[IBIS Ver]   5.1
[File name]   imx8mm_14x14_v1.ibs
[File Rev]   1.0
[Date]   Jan 06,2021
[Notes]   One-Section RLC
[Disclaimer] IMPORTANT NOTICE
  This information is provided on an AS IS basis and without warranty.
  IN NO EVENT SHALL NXP BE LIABLE FOR INCIDENTAL OR CONSEQUENTIAL
  DAMAGES ARISING FROM USE OF THIS INFORMATION. THIS DISCLAIMER OF
  WARRANTY EXTENDS TO THE USER OF THE INFORMATION, AND TO THEIR CUSTOMERS
  OR USERS OF PRODUCTS  AND IS IN LIEU OF ALL WARRANTIES WHETHER EXPRESS,
  IMPLIED, OR STATUTORY, INCLUDING IMPLIED WARRANTIES OF MERCHANTABILITY
  OR FITNESS FOR PARTICULAR PURPOSE.
  NXP does not represent or warrant that the information furnished
  hereunder is free of infringement of any third party patents,
  copyrights, trade secrets, or other intellectual property rights.
  NXP does not represent or warrant that the information is free of
  defect, or that it meets any particular standard, requirements or need
  of the user of the infomation or their customers.
  NXP reserves the right to change the information in this file
  without notice.
   http://www.nxp.com
[Copyright]   (C) Copyright NXP 2007 - 2018, All Rights Reserved.
[Component] imx8mm_14x14_v1.ibs
[Manufacturer] NXP
[Package]
|   typ   min   max
R_pkg   0.37144   0.16325   0.62648
L_pkg   2.82e-9   1.063e-9   4.842e-9
C_pkg   7.818e-13   4.515e-13   1.089e-12
[Pin]   Signal_name   model_name   R_pin   L_pin   C_pin
M19 NVCC_CLK POWER
K8 NVCC_DRAM POWER
K9 NVCC_DRAM POWER
L9 NVCC_DRAM POWER
M9 NVCC_DRAM POWER
N8 NVCC_DRAM POWER
N9 NVCC_DRAM POWER
P7 NVCC_DRAM POWER
R8 NVCC_DRAM POWER
R9 NVCC_DRAM POWER
T9 NVCC_DRAM POWER
U9 NVCC_DRAM POWER
V8 NVCC_DRAM POWER
V9 NVCC_DRAM POWER
H10 NVCC_ECSPI POWER
W22 NVCC_ENET POWER
W12 NVCC_GPIO1 POWER
J11 NVCC_I2C POWER
L19 NVCC_JTAG POWER
U19 NVCC_NAND POWER
W18 NVCC_SAI1 POWER
V19 NVCC_SAI2 POWER
Y10 NVCC_SAI3 POWER
W17 NVCC_SAI5 POWER
V20 NVCC_SD1 POWER
V22 NVCC_SD2 POWER
J22 NVCC_SNVS_1P8 POWER
J12 NVCC_UART POWER
AB13 PVCC0_1P8 POWER
T19 PVCC1_1P8 POWER
J13 PVCC2_1P8 POWER
N19 VDD_24M_XTAL_1P8 POWER
AA14 VDD_ANA0_1P8 POWER
Y15 VDD_ANA0_1P8 POWER
N20 VDD_ANA1_1P8 POWER
P19 VDD_ANA1_1P8 POWER
L17 VDD_ANA_0P8 POWER
N17 VDD_ANA_0P8 POWER
R13 VDD_ARM POWER
R15 VDD_ARM POWER
T13 VDD_ARM POWER
T14 VDD_ARM POWER
T15 VDD_ARM POWER
U13 VDD_ARM POWER
U15 VDD_ARM POWER
V13 VDD_ARM POWER
V15 VDD_ARM POWER
V16 VDD_ARM POWER
W13 VDD_ARM POWER
W14 VDD_ARM POWER
W15 VDD_ARM POWER
W16 VDD_ARM POWER
P16 VDD_ARM_PLL_0P8 POWER
R19 VDD_ARM_PLL_1P8 POWER
J10 VDD_DRAM POWER
L10 VDD_DRAM POWER
N10 VDD_DRAM POWER
R10 VDD_DRAM POWER
U10 VDD_DRAM POWER
W10 VDD_DRAM POWER
P9 VDD_DRAM_PLL_0P8 POWER
P5 VDD_DRAM_PLL_1P8 POWER
P12 VDD_GPU POWER
R11 VDD_GPU POWER
U11 VDD_GPU POWER
V12 VDD_GPU POWER
W11 VDD_GPU POWER
J14 VDD_MIPI_0P9 POWER
J15 VDD_MIPI_1P2 POWER
H13 VDD_MIPI_1P8 POWER
J16 VDD_PCI_0P8 POWER
G14 VDD_PCI_1P8 POWER
K22 VDD_SNVS_0P8 POWER
K15 VDD_SOC POWER
K16 VDD_SOC POWER
L15 VDD_SOC POWER
L18 VDD_SOC POWER
M15 VDD_SOC POWER
N13 VDD_SOC POWER
N15 VDD_SOC POWER
N18 VDD_SOC POWER
R17 VDD_SOC POWER
R18 VDD_SOC POWER
U17 VDD_SOC POWER
U18 VDD_SOC POWER
J17 VDD_USB_0P8 POWER
H15 VDD_USB_1P8 POWER
K19 VDD_USB_3P3 POWER
K12 VDD_VPU POWER
K13 VDD_VPU POWER
L11 VDD_VPU POWER
L13 VDD_VPU POWER
M13 VDD_VPU POWER
M14 VDD_VPU POWER
N11 VDD_VPU POWER
P1 DRAM_VREF POWER
B27 24M_XTALI NC 0.4921 3.82E-09 9.28E-13
C26 24M_XTALO NC 0.45748 3.59E-09 8.46E-13
G26 BOOT_MODE0 PBIDIRHS_E33_33_NT_DR_H 0.38307 3.00E-09 8.24E-13
G27 BOOT_MODE1 PBIDIRHS_E33_33_NT_DR_H 0.40036 3.16E-09 8.38E-13
H27 CLKIN1 PBIDIRHS_E33_33_NT_DR_H 0.36937 3.01E-09 8.01E-13
J27 CLKIN2 PBIDIRHS_E33_33_NT_DR_H 0.4193 3.52E-09 8.49E-13
H26 CLKOUT1 PBIDIRHS_E33_33_NT_DR_H 0.35917 2.90E-09 8.78E-13
J26 CLKOUT2 PBIDIRHS_E33_33_NT_DR_H 0.42161 3.44E-09 8.89E-13
F4 DRAM_AC00 CA_CK 0.42341 3.09E-09 8.52E-13
F5 DRAM_AC01 CA_CK 0.29473 2.13E-09 7.50E-13
K4 DRAM_AC02 CA_CK 0.3399 2.45E-09 5.61E-13
J4 DRAM_AC03 CA_CK 0.36868 2.58E-09 7.56E-13
L2 DRAM_AC04 CA_CK 0.33939 2.34E-09 7.22E-13
L1 DRAM_AC05 CA_CK 0.34212 2.36E-09 7.20E-13
F6 DRAM_AC06 CA_CK 0.34818 2.62E-09 8.00E-13
J5 DRAM_AC07 CA_CK 0.26386 1.87E-09 6.85E-13
J6 DRAM_AC08 CA_CK 0.31308 2.36E-09 6.60E-13
K6 DRAM_AC09 CA_CK 0.20679 1.49E-09 5.66E-13
E4 DRAM_AC10 CA_CK 0.41222 3.00E-09 9.97E-13
D5 DRAM_AC11 CA_CK 0.47769 3.53E-09 1.01E-12
N4 DRAM_AC12 CA_CK 0.24984 1.70E-09 6.69E-13
N5 DRAM_AC13 CA_CK 0.284 1.98E-09 5.24E-13
K5 DRAM_AC14 CA_CK 0.34768 2.50E-09 7.57E-13
N6 DRAM_AC15 CA_CK 0.16325 1.06E-09 4.70E-13
M1 DRAM_AC16 CA_CK 0.31836 2.25E-09 6.88E-13
M2 DRAM_AC17 CA_CK 0.32445 2.22E-09 6.95E-13
N2 DRAM_AC19 CA_CK 0.34499 2.50E-09 7.43E-13
AB4 DRAM_AC20 CA_CK 0.37465 2.80E-09 9.48E-13
AB5 DRAM_AC21 CA_CK 0.38319 2.90E-09 9.15E-13
W4 DRAM_AC22 CA_CK 0.38211 2.84E-09 8.08E-13
V4 DRAM_AC23 CA_CK 0.29471 2.10E-09 7.54E-13
U2 DRAM_AC24 CA_CK 0.34737 2.38E-09 7.32E-13
U1 DRAM_AC25 CA_CK 0.34266 2.43E-09 7.32E-13
N1 DRAM_AC26 CA_CK 0.42632 3.11E-09 9.15E-13
R6 DRAM_AC27 CA_CK 0.22559 1.66E-09 5.07E-13
W6 DRAM_AC28 CA_CK 0.22056 1.60E-09 6.33E-13
V6 DRAM_AC29 CA_CK 0.27799 1.96E-09 6.03E-13
AC4 DRAM_AC30 CA_CK 0.48641 3.58E-09 9.77E-13
AD5 DRAM_AC31 CA_CK 0.41562 3.11E-09 1.02E-12
R4 DRAM_AC32 CA_CK 0.2504 1.78E-09 6.58E-13
R5 DRAM_AC33 CA_CK 0.33425 2.46E-09 6.16E-13
T1 DRAM_AC34 CA_CK 0.321 2.31E-09 7.99E-13
T2 DRAM_AC35 CA_CK 0.42263 2.99E-09 8.89E-13
V5 DRAM_AC36 CA_CK 0.2084 1.47E-09 4.76E-13
W5 DRAM_AC37 CA_CK 0.2624 1.85E-09 6.65E-13
AB6 DRAM_AC38 CA_CK 0.34026 2.47E-09 7.31E-13
R2 DRAM_ALERT_N CA_CK 0.27399 1.90E-09 6.80E-13
A4 DRAM_DM0 DQ_DQS 0.47819 3.40E-09 9.75E-13
F1 DRAM_DM1 DQ_DQS 0.49651 3.45E-09 9.97E-13
AB1 DRAM_DM2 DQ_DQS 0.48699 3.28E-09 8.55E-13
AG4 DRAM_DM3 DQ_DQS 0.43626 2.94E-09 9.57E-13
A5 DRAM_DQ00 DQ_DQS 0.38783 2.72E-09 8.18E-13
B5 DRAM_DQ01 DQ_DQS 0.36282 2.46E-09 7.49E-13
D2 DRAM_DQ02 DQ_DQS 0.4521 3.16E-09 9.42E-13
D1 DRAM_DQ03 DQ_DQS 0.41453 2.88E-09 9.24E-13
C1 DRAM_DQ04 DQ_DQS 0.5585 3.72E-09 9.55E-13
B1 DRAM_DQ05 DQ_DQS 0.50545 3.31E-09 1.01E-12
A3 DRAM_DQ06 DQ_DQS 0.5562 3.84E-09 1.09E-12
B4 DRAM_DQ07 DQ_DQS 0.38982 2.83E-09 9.33E-13
F2 DRAM_DQ08 DQ_DQS 0.38671 2.53E-09 7.96E-13
G2 DRAM_DQ09 DQ_DQS 0.43825 3.05E-09 7.98E-13
J1 DRAM_DQ10 DQ_DQS 0.34914 2.55E-09 8.27E-13
J2 DRAM_DQ11 DQ_DQS 0.40764 2.85E-09 7.90E-13
K2 DRAM_DQ12 DQ_DQS 0.32705 2.20E-09 7.37E-13
K1 DRAM_DQ13 DQ_DQS 0.4328 2.98E-09 8.00E-13
E1 DRAM_DQ14 DQ_DQS 0.43043 3.20E-09 1.07E-12
E2 DRAM_DQ15 DQ_DQS 0.39934 2.85E-09 9.64E-13
AB2 DRAM_DQ16 DQ_DQS 0.39751 2.80E-09 9.41E-13
AA2 DRAM_DQ17 DQ_DQS 0.42671 3.06E-09 8.23E-13
W1 DRAM_DQ18 DQ_DQS 0.45851 3.22E-09 9.25E-13
W2 DRAM_DQ19 DQ_DQS 0.35718 2.37E-09 7.42E-13
V2 DRAM_DQ20 DQ_DQS 0.42378 2.95E-09 9.70E-13
V1 DRAM_DQ21 DQ_DQS 0.40154 2.74E-09 9.04E-13
AC1 DRAM_DQ22 DQ_DQS 0.50433 3.37E-09 8.78E-13
AC2 DRAM_DQ23 DQ_DQS 0.39804 2.61E-09 8.82E-13
AG5 DRAM_DQ24 DQ_DQS 0.50337 3.60E-09 1.01E-12
AF5 DRAM_DQ25 DQ_DQS 0.40676 2.78E-09 9.44E-13
AD2 DRAM_DQ26 DQ_DQS 0.40362 2.64E-09 8.99E-13
AD1 DRAM_DQ27 DQ_DQS 0.51492 3.50E-09 9.36E-13
AE1 DRAM_DQ28 DQ_DQS 0.50761 3.57E-09 9.74E-13
AF1 DRAM_DQ29 DQ_DQS 0.48733 3.31E-09 1.02E-12
AG3 DRAM_DQ30 DQ_DQS 0.38743 2.64E-09 9.43E-13
AF4 DRAM_DQ31 DQ_DQS 0.34632 2.38E-09 8.16E-13
B2 DRAM_DQS0_N DQ_DQS 0.49647 3.43E-09 1.01E-12
A2 DRAM_DQS0_P DQ_DQS 0.49826 3.40E-09 1.01E-12
H1 DRAM_DQS1_N DQ_DQS 0.40732 2.79E-09 8.15E-13
G1 DRAM_DQS1_P DQ_DQS 0.40344 2.79E-09 8.44E-13
Y1 DRAM_DQS2_N DQ_DQS 0.3988 2.81E-09 8.38E-13
AA1 DRAM_DQS2_P DQ_DQS 0.41087 2.86E-09 8.67E-13
AF2 DRAM_DQS3_N DQ_DQS 0.45744 3.20E-09 9.44E-13
AG2 DRAM_DQS3_P DQ_DQS 0.46707 3.23E-09 9.51E-13
R1 DRAM_RESET_N CA_CK 0.29197 2.11E-09 6.87E-13
P2 DRAM_ZN CA_CK 0.24788 1.76E-09 6.75E-13
A7 ECSPI1_MISO PBIDIRHS_E33_33_NT_DR_H 0.38772 2.72E-09 7.65E-13
B7 ECSPI1_MOSI PBIDIRHS_E33_33_NT_DR_H 0.32341 2.35E-09 7.09E-13
D6 ECSPI1_SCLK PBIDIRHS_E33_33_NT_DR_H 0.29275 2.08E-09 7.27E-13
B6 ECSPI1_SS0 PBIDIRHS_E33_33_NT_DR_H 0.35372 2.43E-09 7.80E-13
A8 ECSPI2_MISO PBIDIRHS_E33_33_NT_DR_H 0.40822 3.10E-09 8.51E-13
B8 ECSPI2_MOSI PBIDIRHS_E33_33_NT_DR_H 0.32937 2.39E-09 6.99E-13
E6 ECSPI2_SCLK PBIDIRHS_E33_33_NT_DR_H 0.24697 1.88E-09 5.93E-13
A6 ECSPI2_SS0 PBIDIRHS_E33_33_NT_DR_H 0.40084 2.94E-09 8.99E-13
AC27 ENET_MDC PBIDIRHS_E33_33_NT_DR_H 0.39339 2.87E-09 8.25E-13
AB27 ENET_MDIO PBIDIRHS_E33_33_NT_DR_H 0.46375 3.40E-09 9.21E-13
AE27 ENET_RD0 PBIDIRHS_E33_33_NT_DR_H 0.37558 3.46E-09 8.16E-13
AD27 ENET_RD1 PBIDIRHS_E33_33_NT_DR_H 0.45448 3.87E-09 8.86E-13
AD26 ENET_RD2 PBIDIRHS_E33_33_NT_DR_H 0.40318 3.67E-09 7.77E-13
AC26 ENET_RD3 PBIDIRHS_E33_33_NT_DR_H 0.38258 3.49E-09 7.41E-13
AE26 ENET_RXC PBIDIRHS_E33_33_NT_DR_H 0.40275 3.87E-09 7.29E-13
AF27 ENET_RX_CTL PBIDIRHS_E33_33_NT_DR_H 0.47312 4.13E-09 9.05E-13
AG26 ENET_TD0 PBIDIRHS_E33_33_NT_DR_H 0.56315 4.84E-09 1.05E-12
AF26 ENET_TD1 PBIDIRHS_E33_33_NT_DR_H 0.45897 4.71E-09 8.76E-13
AG25 ENET_TD2 PBIDIRHS_E33_33_NT_DR_H 0.36868 4.20E-09 6.87E-13
AF25 ENET_TD3 PBIDIRHS_E33_33_NT_DR_H 0.43981 3.75E-09 8.85E-13
AG24 ENET_TXC PBIDIRHS_E33_33_NT_DR_H 0.39691 3.64E-09 7.93E-13
AF24 ENET_TX_CTL PBIDIRHS_E33_33_NT_DR_H 0.4156 3.99E-09 8.15E-13
AG14 GPIO1_IO00 PBIDIRHS_E33_33_NT_DR_H 0.38758 3.06E-09 8.41E-13
AF14 GPIO1_IO01 PBIDIRHS_E33_33_NT_DR_H 0.43343 3.44E-09 8.72E-13
AG13 GPIO1_IO02 PBIDIRHS_E33_33_NT_DR_H 0.33948 2.76E-09 7.79E-13
AF13 GPIO1_IO03 PBIDIRHS_E33_33_NT_DR_H 0.35613 2.83E-09 7.48E-13
AG12 GPIO1_IO04 PBIDIRHS_E33_33_NT_DR_H 0.38708 3.02E-09 8.49E-13
AF12 GPIO1_IO05 PBIDIRHS_E33_33_NT_DR_H 0.41325 3.30E-09 8.14E-13
AG11 GPIO1_IO06 PBIDIRHS_E33_33_NT_DR_H 0.31952 2.68E-09 7.33E-13
AF11 GPIO1_IO07 PBIDIRHS_E33_33_NT_DR_H 0.36791 3.03E-09 6.35E-13
AG10 GPIO1_IO08 PBIDIRHS_E33_33_NT_DR_H 0.35936 2.88E-09 8.45E-13
AF10 GPIO1_IO09 PBIDIRHS_E33_33_NT_DR_H 0.41844 3.27E-09 8.04E-13
AD10 GPIO1_IO10 PBIDIRHS_E33_33_NT_DR_H 0.27975 2.23E-09 6.91E-13
AC10 GPIO1_IO11 PBIDIRHS_E33_33_NT_DR_H 0.35499 2.84E-09 7.58E-13
AB10 GPIO1_IO12 PBIDIRHS_E33_33_NT_DR_H 0.23422 1.88E-09 6.06E-13
AD9 GPIO1_IO13 PBIDIRHS_E33_33_NT_DR_H 0.40459 3.14E-09 8.51E-13
AC9 GPIO1_IO14 PBIDIRHS_E33_33_NT_DR_H 0.2988 2.39E-09 7.12E-13
AB9 GPIO1_IO15 PBIDIRHS_E33_33_NT_DR_H 0.36069 2.96E-09 7.56E-13
E9 I2C1_SCL PBIDIRHS_E33_33_NT_DR_H 0.3103 2.52E-09 6.38E-13
F9 I2C1_SDA PBIDIRHS_E33_33_NT_DR_H 0.29328 2.24E-09 5.56E-13
D10 I2C2_SCL PBIDIRHS_E33_33_NT_DR_H 0.33923 2.80E-09 5.75E-13
D9 I2C2_SDA PBIDIRHS_E33_33_NT_DR_H 0.34699 2.80E-09 6.99E-13
E10 I2C3_SCL PBIDIRHS_E33_33_NT_DR_H 0.23391 1.93E-09 5.04E-13
F10 I2C3_SDA PBIDIRHS_E33_33_NT_DR_H 0.1897 1.71E-09 5.05E-13
D13 I2C4_SCL PBIDIRHS_E33_33_NT_DR_H 0.3237 2.64E-09 7.56E-13
E13 I2C4_SDA PBIDIRHS_E33_33_NT_DR_H 0.29041 2.50E-09 6.44E-13
D27 JTAG_MOD PBIDIRHS_E33_33_NT_DR_H 0.55739 4.22E-09 1.07E-12
F26 JTAG_TCK PBIDIRHS_E33_33_NT_DR_H 0.39713 3.13E-09 8.46E-13
E27 JTAG_TDI PBIDIRHS_E33_33_NT_DR_H 0.48323 3.72E-09 9.46E-13
E26 JTAG_TDO PBIDIRHS_E33_33_NT_DR_H 0.46524 3.49E-09 9.61E-13
F27 JTAG_TMS PBIDIRHS_E33_33_NT_DR_H 0.40659 3.20E-09 8.55E-13
C27 JTAG_TRST_B PBIDIRHS_E33_33_NT_DR_H 0.62648 4.65E-09 1.04E-12
A16 MIPI_CSI_CLK_N DPHY_RX 0.3771 2.72E-09 7.60E-13
B16 MIPI_CSI_CLK_P DPHY_RX 0.38283 2.57E-09 7.45E-13
A14 MIPI_CSI_D0_N DPHY_RX 0.37613 2.82E-09 7.79E-13
B14 MIPI_CSI_D0_P DPHY_RX 0.38229 2.82E-09 7.45E-13
A15 MIPI_CSI_D1_N DPHY_RX 0.37466 2.76E-09 7.60E-13
B15 MIPI_CSI_D1_P DPHY_RX 0.38096 2.72E-09 7.41E-13
A17 MIPI_CSI_D2_N DPHY_RX 0.38921 2.64E-09 7.84E-13
B17 MIPI_CSI_D2_P DPHY_RX 0.37689 2.58E-09 7.66E-13
A18 MIPI_CSI_D3_N DPHY_RX 0.38322 2.63E-09 7.91E-13
B18 MIPI_CSI_D3_P DPHY_RX 0.39264 2.70E-09 7.51E-13
A11 MIPI_DSI_CLK_N DPHY_TX 0.37472 2.62E-09 7.87E-13
B11 MIPI_DSI_CLK_P DPHY_TX 0.36236 2.53E-09 7.67E-13
A9 MIPI_DSI_D0_N DPHY_TX 0.38075 2.72E-09 7.96E-13
B9 MIPI_DSI_D0_P DPHY_TX 0.39063 2.78E-09 7.78E-13
A10 MIPI_DSI_D1_N DPHY_TX 0.3757 2.65E-09 7.97E-13
B10 MIPI_DSI_D1_P DPHY_TX 0.38021 2.65E-09 7.54E-13
A12 MIPI_DSI_D2_N DPHY_TX 0.36067 2.56E-09 7.77E-13
B12 MIPI_DSI_D2_P DPHY_TX 0.36995 2.47E-09 7.64E-13
A13 MIPI_DSI_D3_N DPHY_TX 0.36395 2.75E-09 7.63E-13
B13 MIPI_DSI_D3_P DPHY_TX 0.37199 2.72E-09 7.55E-13
D15 MIPI_VREG_CAP NC 0.29573 2.25E-09 6.33E-13
N22 NAND_ALE PBIDIRHS_E33_33_NT_DR_H 0.17446 1.49E-09 4.52E-13
N24 NAND_CE0_B PBIDIRHS_E33_33_NT_DR_H 0.30096 2.52E-09 7.08E-13
P27 NAND_CE1_B PBIDIRHS_E33_33_NT_DR_H 0.31972 2.52E-09 7.03E-13
M27 NAND_CE2_B PBIDIRHS_E33_33_NT_DR_H 0.39508 3.03E-09 7.70E-13
L27 NAND_CE3_B PBIDIRHS_E33_33_NT_DR_H 0.47741 3.76E-09 9.74E-13
K27 NAND_CLE PBIDIRHS_E33_33_NT_DR_H 0.38823 3.12E-09 8.72E-13
P23 NAND_DATA00 PBIDIRHS_E33_33_NT_DR_H 0.28145 2.33E-09 6.02E-13
K24 NAND_DATA01 PBIDIRHS_E33_33_NT_DR_H 0.36133 2.99E-09 7.34E-13
K23 NAND_DATA02 PBIDIRHS_E33_33_NT_DR_H 0.38886 3.16E-09 8.15E-13
N23 NAND_DATA03 PBIDIRHS_E33_33_NT_DR_H 0.28373 2.43E-09 5.87E-13
M26 NAND_DATA04 PBIDIRHS_E33_33_NT_DR_H 0.33508 2.60E-09 7.92E-13
L26 NAND_DATA05 PBIDIRHS_E33_33_NT_DR_H 0.33014 2.62E-09 7.40E-13
K26 NAND_DATA06 PBIDIRHS_E33_33_NT_DR_H 0.39436 3.20E-09 9.12E-13
N26 NAND_DATA07 PBIDIRHS_E33_33_NT_DR_H 0.31059 2.38E-09 6.75E-13
R22 NAND_DQS PBIDIRHS_E33_33_NT_DR_H 0.32581 2.75E-09 6.58E-13
P26 NAND_READY_B PBIDIRHS_E33_33_NT_DR_H 0.35112 2.71E-09 7.06E-13
N27 NAND_RE_B PBIDIRHS_E33_33_NT_DR_H 0.33752 2.66E-09 6.83E-13
R26 NAND_WE_B PBIDIRHS_E33_33_NT_DR_H 0.43434 3.44E-09 8.28E-13
R27 NAND_WP_B PBIDIRHS_E33_33_NT_DR_H 0.42188 3.37E-09 8.14E-13
A25 ONOFF NC 0.43844 3.19E-09 8.95E-13
A21 PCIE_CLK_N TX_TOP 0.33922 2.64E-09 8.40E-13
B21 PCIE_CLK_P TX_TOP 0.329 2.52E-09 8.65E-13
D19 PCIE_RESREF NC 0.2402 2.15E-09 6.74E-13
A19 PCIE_RXN_N NC 0.28475 2.21E-09 7.35E-13
B19 PCIE_RXN_P NC 0.29669 2.19E-09 7.64E-13
A20 PCIE_TXN_N TX_TOP 0.30756 2.39E-09 7.71E-13
B20 PCIE_TXN_P TX_TOP 0.3233 2.40E-09 7.90E-13
A24 PMIC_ON_REQ PBIDIR_E33_33_FS_DR_H 0.4719 3.40E-09 8.55E-13
E24 PMIC_STBY_REQ PBIDIR_E33_33_FS_DR_H 0.32278 2.45E-09 6.19E-13
B24 POR_B NC 0.42336 3.21E-09 8.44E-13
F24 RTC_RESET_B NC 0.29975 2.34E-09 6.38E-13
A26 RTC_XTALI NC 0.50151 3.83E-09 9.40E-13
B25 RTC_XTALO NC 0.46144 3.53E-09 8.96E-13
AB18 SAI1_MCLK PBIDIRHS_E33_33_NT_DR_H 0.20397 1.67E-09 5.25E-13
AF16 SAI1_RXC PBIDIRHS_E33_33_NT_DR_H 0.3861 3.04E-09 7.41E-13
AG15 SAI1_RXD0 PBIDIRHS_E33_33_NT_DR_H 0.37411 2.91E-09 8.55E-13
AF15 SAI1_RXD1 PBIDIRHS_E33_33_NT_DR_H 0.40099 3.10E-09 7.70E-13
AG17 SAI1_RXD2 PBIDIRHS_E33_33_NT_DR_H 0.38437 2.98E-09 8.23E-13
AF17 SAI1_RXD3 PBIDIRHS_E33_33_NT_DR_H 0.40145 3.10E-09 7.97E-13
AG18 SAI1_RXD4 PBIDIRHS_E33_33_NT_DR_H 0.40491 3.16E-09 8.75E-13
AF18 SAI1_RXD5 PBIDIRHS_E33_33_NT_DR_H 0.43013 3.31E-09 8.09E-13
AG19 SAI1_RXD6 PBIDIRHS_E33_33_NT_DR_H 0.37629 2.87E-09 7.63E-13
AF19 SAI1_RXD7 PBIDIRHS_E33_33_NT_DR_H 0.426 3.22E-09 7.84E-13
AG16 SAI1_RXFS PBIDIRHS_E33_33_NT_DR_H 0.34355 2.65E-09 7.51E-13
AC18 SAI1_TXC PBIDIRHS_E33_33_NT_DR_H 0.25163 2.00E-09 5.74E-13
AG20 SAI1_TXD0 PBIDIRHS_E33_33_NT_DR_H 0.45434 3.52E-09 8.66E-13
AF20 SAI1_TXD1 PBIDIRHS_E33_33_NT_DR_H 0.38925 2.98E-09 8.30E-13
AG21 SAI1_TXD2 PBIDIRHS_E33_33_NT_DR_H 0.48048 3.62E-09 9.03E-13
AF21 SAI1_TXD3 PBIDIRHS_E33_33_NT_DR_H 0.41011 3.08E-09 7.74E-13
AG22 SAI1_TXD4 PBIDIRHS_E33_33_NT_DR_H 0.50267 3.75E-09 9.02E-13
AF22 SAI1_TXD5 PBIDIRHS_E33_33_NT_DR_H 0.39677 2.92E-09 8.01E-13
AG23 SAI1_TXD6 PBIDIRHS_E33_33_NT_DR_H 0.48107 3.54E-09 8.85E-13
AF23 SAI1_TXD7 PBIDIRHS_E33_33_NT_DR_H 0.47026 3.42E-09 9.22E-13
AB19 SAI1_TXFS PBIDIRHS_E33_33_NT_DR_H 0.33879 2.72E-09 6.75E-13
AD19 SAI2_MCLK PBIDIRHS_E33_33_NT_DR_H 0.34927 2.71E-09 7.35E-13
AB22 SAI2_RXC PBIDIRHS_E33_33_NT_DR_H 0.39152 3.22E-09 6.96E-13
AC24 SAI2_RXD0 PBIDIRHS_E33_33_NT_DR_H 0.47686 3.99E-09 7.79E-13
AC19 SAI2_RXFS PBIDIRHS_E33_33_NT_DR_H 0.41406 3.11E-09 7.52E-13
AD22 SAI2_TXC PBIDIRHS_E33_33_NT_DR_H 0.39577 2.91E-09 6.81E-13
AC22 SAI2_TXD0 PBIDIRHS_E33_33_NT_DR_H 0.4 3.28E-09 7.17E-13
AD23 SAI2_TXFS PBIDIRHS_E33_33_NT_DR_H 0.49896 3.72E-09 8.77E-13
AD6 SAI3_MCLK PBIDIRHS_E33_33_NT_DR_H 0.29662 2.07E-09 7.13E-13
AG7 SAI3_RXC PBIDIRHS_E33_33_NT_DR_H 0.35957 2.55E-09 8.65E-13
AF7 SAI3_RXD PBIDIRHS_E33_33_NT_DR_H 0.35325 2.61E-09 7.82E-13
AG8 SAI3_RXFS PBIDIRHS_E33_33_NT_DR_H 0.33908 2.41E-09 7.81E-13
AG6 SAI3_TXC PBIDIRHS_E33_33_NT_DR_H 0.3654 2.55E-09 8.74E-13
AF6 SAI3_TXD PBIDIRHS_E33_33_NT_DR_H 0.33587 2.26E-09 7.83E-13
AC6 SAI3_TXFS PBIDIRHS_E33_33_NT_DR_H 0.30575 2.39E-09 7.29E-13
AD15 SAI5_MCLK PBIDIRHS_E33_33_NT_DR_H 0.25675 2.05E-09 6.62E-13
AC15 SAI5_RXC PBIDIRHS_E33_33_NT_DR_H 0.28559 2.32E-09 5.94E-13
AD18 SAI5_RXD0 PBIDIRHS_E33_33_NT_DR_H 0.34056 2.66E-09 7.86E-13
AC14 SAI5_RXD1 PBIDIRHS_E33_33_NT_DR_H 0.2822 2.24E-09 5.55E-13
AD13 SAI5_RXD2 PBIDIRHS_E33_33_NT_DR_H 0.26671 2.07E-09 6.33E-13
AC13 SAI5_RXD3 PBIDIRHS_E33_33_NT_DR_H 0.30639 2.47E-09 6.36E-13
AB15 SAI5_RXFS PBIDIRHS_E33_33_NT_DR_H 0.20336 1.68E-09 5.65E-13
V26 SD1_CLK PBIDIRHS_E33_33_NT_DR_H 0.33244 2.62E-09 6.79E-13
V27 SD1_CMD PBIDIRHS_E33_33_NT_DR_H 0.43797 3.69E-09 7.76E-13
Y27 SD1_DATA0 PBIDIRHS_E33_33_NT_DR_H 0.43231 3.54E-09 9.74E-13
Y26 SD1_DATA1 PBIDIRHS_E33_33_NT_DR_H 0.48715 3.96E-09 1.00E-12
T27 SD1_DATA2 PBIDIRHS_E33_33_NT_DR_H 0.34183 2.77E-09 7.27E-13
T26 SD1_DATA3 PBIDIRHS_E33_33_NT_DR_H 0.3745 3.05E-09 7.07E-13
U27 SD1_DATA4 PBIDIRHS_E33_33_NT_DR_H 0.40399 3.25E-09 7.74E-13
U26 SD1_DATA5 PBIDIRHS_E33_33_NT_DR_H 0.2998 2.59E-09 6.84E-13
W27 SD1_DATA6 PBIDIRHS_E33_33_NT_DR_H 0.36633 3.12E-09 7.00E-13
W26 SD1_DATA7 PBIDIRHS_E33_33_NT_DR_H 0.46231 3.79E-09 9.16E-13
R23 SD1_RESET_B PBIDIRHS_E33_33_NT_DR_H 0.23368 2.06E-09 5.55E-13
R24 SD1_STROBE PBIDIRHS_E33_33_NT_DR_H 0.36755 3.16E-09 6.72E-13
AA26 SD2_CD_B PBIDIRHS_E33_33_NT_DR_H 0.3582 2.82E-09 7.71E-13
W23 SD2_CLK PBIDIRHS_E33_33_NT_DR_H 0.31294 2.58E-09 6.06E-13
W24 SD2_CMD PBIDIRHS_E33_33_NT_DR_H 0.28036 2.25E-09 5.54E-13
AB23 SD2_DATA0 PBIDIRHS_E33_33_NT_DR_H 0.36202 2.91E-09 6.66E-13
AB24 SD2_DATA1 PBIDIRHS_E33_33_NT_DR_H 0.39937 3.19E-09 8.23E-13
V24 SD2_DATA2 PBIDIRHS_E33_33_NT_DR_H 0.33753 2.81E-09 5.66E-13
V23 SD2_DATA3 PBIDIRHS_E33_33_NT_DR_H 0.20962 1.82E-09 5.07E-13
AB26 SD2_RESET_B PBIDIRHS_E33_33_NT_DR_H 0.40769 3.12E-09 7.65E-13
AA27 SD2_WP PBIDIRHS_E33_33_NT_DR_H 0.44218 3.59E-09 8.17E-13
AF8 SPDIF_EXT_CLK PBIDIRHS_E33_33_NT_DR_H 0.32482 2.17E-09 6.91E-13
AG9 SPDIF_RX PBIDIRHS_E33_33_NT_DR_H 0.35355 2.50E-09 7.76E-13
AF9 SPDIF_TX PBIDIRHS_E33_33_NT_DR_H 0.32893 2.48E-09 6.63E-13
D26 TEST_MODE PBIDIRHS_E33_33_NT_DR_H 0.50042 4.00E-09 9.69E-13
J24 TSENSOR_RES_EXT NC 0.36131 3.05E-09 6.97E-13
J23 TSENSOR_TEST_OUT NC 0.337 2.88E-09 5.61E-13
E14 UART1_RXD PBIDIRHS_E33_33_NT_DR_H 0.25669 2.16E-09 6.53E-13
F13 UART1_TXD PBIDIRHS_E33_33_NT_DR_H 0.1869 1.69E-09 4.78E-13
F15 UART2_RXD PBIDIRHS_E33_33_NT_DR_H 0.22006 1.99E-09 5.83E-13
E15 UART2_TXD PBIDIRHS_E33_33_NT_DR_H 0.33535 2.69E-09 7.63E-13
E18 UART3_RXD PBIDIRHS_E33_33_NT_DR_H 0.40711 3.32E-09 8.54E-13
D18 UART3_TXD PBIDIRHS_E33_33_NT_DR_H 0.50146 4.01E-09 9.84E-13
F19 UART4_RXD PBIDIRHS_E33_33_NT_DR_H 0.37271 3.21E-09 8.27E-13
F18 UART4_TXD PBIDIRHS_E33_33_NT_DR_H 0.40719 3.37E-09 8.80E-13
A22 USB1_DN USB2_HS_IBIS 0.35212 2.71E-09 8.53E-13
B22 USB1_DP USB2_HS_IBIS 0.3559 2.70E-09 8.34E-13
D22 USB1_ID NC 0.35782 2.49E-09 7.76E-13
E19 USB1_TXRTUNE NC 0.25007 1.71E-09 6.02E-13
F22 USB1_VBUS NC 0.31112 2.14E-09 7.03E-13
A23 USB2_DN USB2_HS_IBIS 0.37213 2.79E-09 8.74E-13
B23 USB2_DP USB2_HS_IBIS 0.37247 2.81E-09 8.43E-13
D23 USB2_ID NC 0.35045 2.42E-09 7.83E-13
E22 USB2_TXRTUNE NC 0.28604 2.02E-09 6.44E-13
F23 USB2_VBUS NC 0.30942 2.17E-09 7.25E-13
A1 VSS GND
A27 VSS GND
AA7 VSS GND
AA9 VSS GND
AA10 VSS GND
AA13 VSS GND
AA15 VSS GND
AA18 VSS GND
AA19 VSS GND
AA21 VSS GND
AB3 VSS GND
AB25 VSS GND
AC3 VSS GND
AC25 VSS GND
AE2 VSS GND
AE5 VSS GND
AE6 VSS GND
AE9 VSS GND
AE10 VSS GND
AE13 VSS GND
AE14 VSS GND
AE15 VSS GND
AE18 VSS GND
AE19 VSS GND
AE22 VSS GND
AE23 VSS GND
AF3 VSS GND
AG1 VSS GND
AG27 VSS GND
B3 VSS GND
B26 VSS GND
C2 VSS GND
C5 VSS GND
C6 VSS GND
C9 VSS GND
C10 VSS GND
C13 VSS GND
C14 VSS GND
C15 VSS GND
C18 VSS GND
C19 VSS GND
C22 VSS GND
C23 VSS GND
E3 VSS GND
E25 VSS GND
F3 VSS GND
F25 VSS GND
G7 VSS GND
G9 VSS GND
G10 VSS GND
G13 VSS GND
G15 VSS GND
G18 VSS GND
G19 VSS GND
G21 VSS GND
H2 VSS GND
H18 VSS GND
J3 VSS GND
J7 VSS GND
J21 VSS GND
J25 VSS GND
K3 VSS GND
K7 VSS GND
K20 VSS GND
K21 VSS GND
K25 VSS GND
L12 VSS GND
L16 VSS GND
M12 VSS GND
M16 VSS GND
N3 VSS GND
N7 VSS GND
N12 VSS GND
N16 VSS GND
N21 VSS GND
N25 VSS GND
P3 VSS GND
P13 VSS GND
P15 VSS GND
P21 VSS GND
P25 VSS GND
R3 VSS GND
R7 VSS GND
R12 VSS GND
R16 VSS GND
R20 VSS GND
R21 VSS GND
R25 VSS GND
T12 VSS GND
T16 VSS GND
U12 VSS GND
U16 VSS GND
V3 VSS GND
V7 VSS GND
V21 VSS GND
V25 VSS GND
W3 VSS GND
W7 VSS GND
W21 VSS GND
W25 VSS GND
Y2 VSS GND
Y13 VSS GND
Y18 VSS GND
[Diff_pin] inv_pin vdiff tdelay_typ tdelay_min tdelay_max
L2 L1 0.140V 0ns NA NA
M1 M2 0.140V 0ns NA NA
AB4 AB5 0.140V 0ns NA NA
U2 U1 0.140V 0ns NA NA
A2 B2 0.140V 0ns NA NA
G1 H1 0.140V 0ns NA NA
AA1 Y1 0.140V 0ns NA NA
AG2 AF2 0.140V 0ns NA NA
B16 A16 NA NA NA NA
B14 A14 NA NA NA NA
B15 A15 NA NA NA NA
B17 A17 NA NA NA NA
B18 A18 NA NA NA NA
B11 A11 NA NA NA NA
B9 A9 NA NA NA NA
B10 A10 NA NA NA NA
B12 A12 NA NA NA NA
B13 A13 NA NA NA NA
B21 A21 NA NA NA NA
B19 A19 NA NA NA NA
B20 A20 NA NA NA NA
B22 A22 150.000mV 0ns NA NA
B23 A23 150.000mV 0ns NA NA
[Model Selector] DQ_DQS
mal4drv27_d3_28   DDR3 mal4drv27 cell  Z0=28-Ohm Driver
mal4drv27_d3_34   DDR3 mal4drv27 cell  Z0=34-Ohm Driver
mal4drv27_d3_40   DDR3 mal4drv27 cell  Z0=40-Ohm Driver
mal4drv27_d3_53   DDR3 mal4drv27 cell  Z0=53-Ohm Driver
mal4drv27_d3_60   DDR3 mal4drv27 cell  Z0=60-Ohm Driver
mal4drv27_d3_odt120   DDR3 mal4drv27 cell 120-Ohm ODT Receiver
mal4drv27_d3_odt60   DDR3 mal4drv27 cell 60-Ohm ODT Receiver
mal4drv27_d3l_28   DDR3L mal4drv27 cell  Z0=28-Ohm Driver
mal4drv27_d3l_34   DDR3L mal4drv27 cell  Z0=34-Ohm Driver
mal4drv27_d3l_40   DDR3L mal4drv27 cell  Z0=40-Ohm Driver
mal4drv27_d3l_53   DDR3L mal4drv27 cell  Z0=53-Ohm Driver
mal4drv27_d3l_60   DDR3L mal4drv27 cell  Z0=60-Ohm Driver
mal4drv27_d3l_odt120   DDR3L mal4drv27 cell 120-Ohm ODT Receiver
mal4drv27_d3l_odt60   DDR3L mal4drv27 cell 60-Ohm ODT Receiver
mal4drv27_d4_28   DDR4 mal4drv27 cell  Z0=28-Ohm Driver
mal4drv27_d4_34   DDR4 mal4drv27 cell  Z0=34-Ohm Driver
mal4drv27_d4_40   DDR4 mal4drv27 cell  Z0=40-Ohm Driver
mal4drv27_d4_53   DDR4 mal4drv27 cell  Z0=53-Ohm Driver
mal4drv27_d4_60   DDR4 mal4drv27 cell  Z0=60-Ohm Driver
mal4drv27_d4_odt120   DDR4 mal4drv27 cell 120-Ohm ODT Receiver
mal4drv27_d4_odt240   DDR4 mal4drv27 cell 240-Ohm ODT Receiver
mal4drv27_d4_odt48   DDR4 mal4drv27 cell 48-Ohm ODT Receiver
mal4drv27_d4_odt60   DDR4 mal4drv27 cell 60-Ohm ODT Receiver
mal4drv27_d4_odt80   DDR4 mal4drv27 cell 80-Ohm ODT Receiver
mal4drv27_dl4_28   LPDDR4 mal4drv27 cell  Z0=28-Ohm Driver
mal4drv27_dl4_34   LPDDR4 mal4drv27 cell  Z0=34-Ohm Driver
mal4drv27_dl4_40   LPDDR4 mal4drv27 cell  Z0=40-Ohm Driver
mal4drv27_dl4_53   LPDDR4 mal4drv27 cell  Z0=53-Ohm Driver
mal4drv27_dl4_60   LPDDR4 mal4drv27 cell  Z0=60-Ohm Driver
mal4drv27_dl4_odt48   LPDDR4 mal4drv27 cell 48-Ohm ODT Receiver
mal4drv27_dl4_odt60   LPDDR4 mal4drv27 cell 60-Ohm ODT Receiver
[Model Selector] CA_CK
mal4drv20_d3_20   DDR3 mal4drv20 cell  Z0=20-Ohm Driver
mal4drv20_d3_24   DDR3 mal4drv20 cell  Z0=24-Ohm Driver
mal4drv20_d3_30   DDR3 mal4drv20 cell  Z0=30-Ohm Driver
mal4drv20_d3_40   DDR3 mal4drv20 cell  Z0=40-Ohm Driver
mal4drv20_d3_60   DDR3 mal4drv20 cell  Z0=60-Ohm Driver
mal4drv20_d3l_20   DDR3L mal4drv20 cell  Z0=20-Ohm Driver
mal4drv20_d3l_24   DDR3L mal4drv20 cell  Z0=24-Ohm Driver
mal4drv20_d3l_30   DDR3L mal4drv20 cell  Z0=30-Ohm Driver
mal4drv20_d3l_40   DDR3L mal4drv20 cell  Z0=40-Ohm Driver
mal4drv20_d3l_60   DDR3L mal4drv20 cell  Z0=60-Ohm Driver
mal4drv20_d4_20   DDR4 mal4drv20 cell  Z0=20-Ohm Driver
mal4drv20_d4_24   DDR4 mal4drv20 cell  Z0=24-Ohm Driver
mal4drv20_d4_30   DDR4 mal4drv20 cell  Z0=30-Ohm Driver
mal4drv20_d4_40   DDR4 mal4drv20 cell  Z0=40-Ohm Driver
mal4drv20_d4_60   DDR4 mal4drv20 cell  Z0=60-Ohm Driver
mal4drv20_dl4_20   LPDDR4 mal4drv20 cell  Z0=20-Ohm Driver
mal4drv20_dl4_24   LPDDR4 mal4drv20 cell  Z0=24-Ohm Driver
mal4drv20_dl4_30   LPDDR4 mal4drv20 cell  Z0=30-Ohm Driver
mal4drv20_dl4_40   LPDDR4 mal4drv20 cell  Z0=40-Ohm Driver
mal4drv20_dl4_60   LPDDR4 mal4drv20 cell  Z0=60-Ohm Driver
[Model Selector] TX_TOP
TX_TOP_32BIT_FAST_HT_HV  32BIT_FAST_HT_HV
TX_TOP_32BIT_SLOW_LT_LV  32BIT_SLOW_LT_LV
TX_TOP_32BIT_TYPICAL   32BIT_TYPICAL
TX_TOP_64BIT_FAST_HT_HV  64BIT_FAST_HT_HV
TX_TOP_64BIT_SLOW_LT_LV  64BIT_SLOW_LT_LV
TX_TOP_64BIT_TYPICAL   64BIT_TYPICAL
[Model Selector] USB2_HS_IBIS
USB2_HSRX   USB2 HS RX model
USB2_HSTX_00_0_01_0011_11   USB2 HS TX model: AMP_PULSE_RISE_VREF_XV=00_0_01_0011_11
[Model Selector] PBIDIR_E33_33_FS_DR_H
| Model Description
M0_PBIDIR_FS_DR_02_1P80V   - 2mA drive strength, fast output slew: - without weak pull
M1_PBIDIR_FS_DR_02_1P80V   - 2mA drive strength, fast output slew: - with weak pulldown
M2_PBIDIR_FS_DR_02_1P80V   - 2mA drive strength, fast output slew: - with weak pullup
M3_PBIDIR_FS_DR_02_1P80V   - 2mA drive strength, slow output slew: - without weak pull
M4_PBIDIR_FS_DR_02_1P80V   - 2mA drive strength, slow output slew: - with weak pulldown
M5_PBIDIR_FS_DR_02_1P80V   - 2mA drive strength, slow output slew: - with weak pullup
M6_PBIDIR_FS_DR_04_1P80V   - 4mA drive strength, fast output slew: - without weak pull
M7_PBIDIR_FS_DR_04_1P80V   - 4mA drive strength, fast output slew: - with weak pulldown
M8_PBIDIR_FS_DR_04_1P80V   - 4mA drive strength, fast output slew: - with weak pullup
M9_PBIDIR_FS_DR_04_1P80V   - 4mA drive strength, slow output slew: - without weak pull
M10_PBIDIR_FS_DR_0_1P80V   - 4mA drive strength, slow output slew: - with weak pulldown
M11_PBIDIR_FS_DR_0_1P80V   - 4mA drive strength, slow output slew: - with weak pullup
M12_PBIDIR_FS_DR_0_1P80V   - 8mA drive strength, fast output slew: - without weak pull
M13_PBIDIR_FS_DR_0_1P80V   - 8mA drive strength, fast output slew: - with weak pulldown
M14_PBIDIR_FS_DR_0_1P80V   - 8mA drive strength, fast output slew: - with weak pullup
M15_PBIDIR_FS_DR_0_1P80V   - 8mA drive strength, slow output slew: - without weak pull
M16_PBIDIR_FS_DR_0_1P80V   - 8mA drive strength, slow output slew: - with weak pulldown
M17_PBIDIR_FS_DR_0_1P80V   - 8mA drive strength, slow output slew: - with weak pullup
M18_PBIDIR_FS_DR_1_1P80V   - 12mA drive strength, fast output slew: - without weak pull
M19_PBIDIR_FS_DR_1_1P80V   - 12mA drive strength, fast output slew: - with weak pulldown
M20_PBIDIR_FS_DR_1_1P80V   - 12mA drive strength, fast output slew: - with weak pullup
M21_PBIDIR_FS_DR_1_1P80V   - 12mA drive strength, slow output slew: - without weak pull
M22_PBIDIR_FS_DR_1_1P80V   - 12mA drive strength, slow output slew: - with weak pulldown
M23_PBIDIR_FS_DR_1_1P80V   - 12mA drive strength, slow output slew: - with weak pullup
M0_PBIDIR_FS_DR_02_3P30V   - 2mA drive strength, fast output slew: - without weak pull
M1_PBIDIR_FS_DR_02_3P30V   - 2mA drive strength, fast output slew: - with weak pulldown
M2_PBIDIR_FS_DR_02_3P30V   - 2mA drive strength, fast output slew: - with weak pullup
M3_PBIDIR_FS_DR_02_3P30V   - 2mA drive strength, slow output slew: - without weak pull
M4_PBIDIR_FS_DR_02_3P30V   - 2mA drive strength, slow output slew: - with weak pulldown
M5_PBIDIR_FS_DR_02_3P30V   - 2mA drive strength, slow output slew: - with weak pullup
M6_PBIDIR_FS_DR_04_3P30V   - 4mA drive strength, fast output slew: - without weak pull
M7_PBIDIR_FS_DR_04_3P30V   - 4mA drive strength, fast output slew: - with weak pulldown
M8_PBIDIR_FS_DR_04_3P30V   - 4mA drive strength, fast output slew: - with weak pullup
M9_PBIDIR_FS_DR_04_3P30V   - 4mA drive strength, slow output slew: - without weak pull
M10_PBIDIR_FS_DR_0_3P30V   - 4mA drive strength, slow output slew: - with weak pulldown
M11_PBIDIR_FS_DR_0_3P30V   - 4mA drive strength, slow output slew: - with weak pullup
M12_PBIDIR_FS_DR_0_3P30V   - 8mA drive strength, fast output slew: - without weak pull
M13_PBIDIR_FS_DR_0_3P30V   - 8mA drive strength, fast output slew: - with weak pulldown
M14_PBIDIR_FS_DR_0_3P30V   - 8mA drive strength, fast output slew: - with weak pullup
M15_PBIDIR_FS_DR_0_3P30V   - 8mA drive strength, slow output slew: - without weak pull
M16_PBIDIR_FS_DR_0_3P30V   - 8mA drive strength, slow output slew: - with weak pulldown
M17_PBIDIR_FS_DR_0_3P30V   - 8mA drive strength, slow output slew: - with weak pullup
M18_PBIDIR_FS_DR_1_3P30V   - 12mA drive strength, fast output slew: - without weak pull
M19_PBIDIR_FS_DR_1_3P30V   - 12mA drive strength, fast output slew: - with weak pulldown
M20_PBIDIR_FS_DR_1_3P30V   - 12mA drive strength, fast output slew: - with weak pullup
M21_PBIDIR_FS_DR_1_3P30V   - 12mA drive strength, slow output slew: - without weak pull
M22_PBIDIR_FS_DR_1_3P30V   - 12mA drive strength, slow output slew: - with weak pulldown
M23_PBIDIR_FS_DR_1_3P30V   - 12mA drive strength, slow output slew: - with weak pullup
[Model Selector] PBIDIRHS_E33_33_NT_DR_H
| Model Description
M0_PBIDIR_HS_02_F_1P80V   - 2mA drive strength, fast output slew: - without weak pull
M1_PBIDIR_HS_02_F_1P80V   - 2mA drive strength, fast output slew: - with weak pulldown
M2_PBIDIR_HS_02_F_1P80V   - 2mA drive strength, fast output slew: - with weak pullup
M3_PBIDIR_HS_02_S_1P80V   - 2mA drive strength, slow output slew: - without weak pull
M4_PBIDIR_HS_02_S_1P80V   - 2mA drive strength, slow output slew: - with weak pulldown
M5_PBIDIR_HS_02_S_1P80V   - 2mA drive strength, slow output slew: - with weak pullup
M6_PBIDIR_HS_04_F_1P80V   - 4mA drive strength, fast output slew: - without weak pull
M7_PBIDIR_HS_04_F_1P80V   - 4mA drive strength, fast output slew: - with weak pulldown
M8_PBIDIR_HS_04_F_1P80V   - 4mA drive strength, fast output slew: - with weak pullup
M9_PBIDIR_HS_04_S_1P80V   - 4mA drive strength, slow output slew: - without weak pull
M10_PBIDIR_HS_04_S_1P80V   - 4mA drive strength, slow output slew: - with weak pulldown
M11_PBIDIR_HS_04_S_1P80V   - 4mA drive strength, slow output slew: - with weak pullup
M12_PBIDIR_HS_08_F_1P80V   - 8mA drive strength, fast output slew: - without weak pull
M13_PBIDIR_HS_08_F_1P80V   - 8mA drive strength, fast output slew: - with weak pulldown
M14_PBIDIR_HS_08_F_1P80V   - 8mA drive strength, fast output slew: - with weak pullup
M15_PBIDIR_HS_08_S_1P80V   - 8mA drive strength, slow output slew: - without weak pull
M16_PBIDIR_HS_08_S_1P80V   - 8mA drive strength, slow output slew: - with weak pulldown
M17_PBIDIR_HS_08_S_1P80V   - 8mA drive strength, slow output slew: - with weak pullup
M18_PBIDIR_HS_12_F_1P80V   - 12mA drive strength, fast output slew: - without weak pull
M19_PBIDIR_HS_12_F_1P80V   - 12mA drive strength, fast output slew: - with weak pulldown
M20_PBIDIR_HS_12_F_1P80V   - 12mA drive strength, fast output slew: - with weak pullup
M21_PBIDIR_HS_12_S_1P80V   - 12mA drive strength, slow output slew: - without weak pull
M22_PBIDIR_HS_12_S_1P80V   - 12mA drive strength, slow output slew: - with weak pulldown
M23_PBIDIR_HS_12_S_1P80V   - 12mA drive strength, slow output slew: - with weak pullup
M0_PBIDIR_HS_02_F_3P30V   - 2mA drive strength, fast output slew: - without weak pull
M1_PBIDIR_HS_02_F_3P30V   - 2mA drive strength, fast output slew: - with weak pulldown
M2_PBIDIR_HS_02_F_3P30V   - 2mA drive strength, fast output slew: - with weak pullup
M3_PBIDIR_HS_02_S_3P30V   - 2mA drive strength, slow output slew: - without weak pull
M4_PBIDIR_HS_02_S_3P30V   - 2mA drive strength, slow output slew: - with weak pulldown
M5_PBIDIR_HS_02_S_3P30V   - 2mA drive strength, slow output slew: - with weak pullup
M6_PBIDIR_HS_04_F_3P30V   - 4mA drive strength, fast output slew: - without weak pull
M7_PBIDIR_HS_04_F_3P30V   - 4mA drive strength, fast output slew: - with weak pulldown
M8_PBIDIR_HS_04_F_3P30V   - 4mA drive strength, fast output slew: - with weak pullup
M9_PBIDIR_HS_04_S_3P30V   - 4mA drive strength, slow output slew: - without weak pull
M10_PBIDIR_HS_04_S_3P30V   - 4mA drive strength, slow output slew: - with weak pulldown
M11_PBIDIR_HS_04_S_3P30V   - 4mA drive strength, slow output slew: - with weak pullup
M12_PBIDIR_HS_08_F_3P30V   - 8mA drive strength, fast output slew: - without weak pull
M13_PBIDIR_HS_08_F_3P30V   - 8mA drive strength, fast output slew: - with weak pulldown
M14_PBIDIR_HS_08_F_3P30V   - 8mA drive strength, fast output slew: - with weak pullup
M15_PBIDIR_HS_08_S_3P30V   - 8mA drive strength, slow output slew: - without weak pull
M16_PBIDIR_HS_08_S_3P30V   - 8mA drive strength, slow output slew: - with weak pulldown
M17_PBIDIR_HS_08_S_3P30V   - 8mA drive strength, slow output slew: - with weak pullup
M18_PBIDIR_HS_12_F_3P30V   - 12mA drive strength, fast output slew: - without weak pull
M19_PBIDIR_HS_12_F_3P30V   - 12mA drive strength, fast output slew: - with weak pulldown
M20_PBIDIR_HS_12_F_3P30V   - 12mA drive strength, fast output slew: - with weak pullup
M21_PBIDIR_HS_12_S_3P30V   - 12mA drive strength, slow output slew: - without weak pull
M22_PBIDIR_HS_12_S_3P30V   - 12mA drive strength, slow output slew: - with weak pulldown
M23_PBIDIR_HS_12_S_3P30V   - 12mA drive strength, slow output slew: - with weak pullup
| Models and submodels in the file (221): mal4drv27_d3_28 (I/O), mal4drv27_d3_34 (I/O), mal4drv27_d3_40 (I/O), mal4drv27_d3_53 (I/O), mal4drv27_d3_60 (I/O), mal4drv27_d3_odt120 (Input), mal4drv27_d3_odt60 (Input), mal4drv27_d3l_28 (I/O), mal4drv27_d3l_34 (I/O), mal4drv27_d3l_40 (I/O), mal4drv27_d3l_53 (I/O), mal4drv27_d3l_60 (I/O), mal4drv27_d3l_odt120 (Input), mal4drv27_d3l_odt60 (Input), mal4drv27_d4_28 (I/O), mal4drv27_d4_34 (I/O), mal4drv27_d4_40 (I/O), mal4drv27_d4_53 (I/O), mal4drv27_d4_60 (I/O), mal4drv27_d4_odt120 (Input), mal4drv27_d4_odt240 (Input), mal4drv27_d4_odt48 (Input), mal4drv27_d4_odt60 (Input), mal4drv27_d4_odt80 (Input), mal4drv27_dl4_28 (I/O), mal4drv27_dl4_34 (I/O), mal4drv27_dl4_40 (I/O), mal4drv27_dl4_53 (I/O), mal4drv27_dl4_60 (I/O), mal4drv27_dl4_odt48 (Input), mal4drv27_dl4_odt60 (Input), mal4drv20_d3_20 (I/O), mal4drv20_d3_24 (I/O), mal4drv20_d3_30 (I/O), mal4drv20_d3_40 (I/O), mal4drv20_d3_60 (I/O), mal4drv20_d3l_20 (I/O), mal4drv20_d3l_24 (I/O), mal4drv20_d3l_30 (I/O), mal4drv20_d3l_40 (I/O), mal4drv20_d3l_60 (I/O), mal4drv20_d4_20 (I/O), mal4drv20_d4_24 (I/O), mal4drv20_d4_30 (I/O), mal4drv20_d4_40 (I/O), mal4drv20_d4_60 (I/O), mal4drv20_dl4_20 (I/O), mal4drv20_dl4_24 (I/O), mal4drv20_dl4_30 (I/O), mal4drv20_dl4_40 (I/O), mal4drv20_dl4_60 (I/O), DPHY_TX (Output), DPHY_RX (Input), TX_TOP_32BIT_FAST_HT_HV (Output), TX_TOP_32BIT_SLOW_LT_LV (Output), TX_TOP_32BIT_TYPICAL (Output), TX_TOP_64BIT_FAST_HT_HV (Output), TX_TOP_64BIT_SLOW_LT_LV (Output), TX_TOP_64BIT_TYPICAL (Output), M0_PBIDIR_FS_DR_02_1P80V (I/O), M1_PBIDIR_FS_DR_02_1P80V (I/O), M1_PBIDIR_FS_DR_02_1P80V_T (Dynamic_clamp), M2_PBIDIR_FS_DR_02_1P80V (I/O), M2_PBIDIR_FS_DR_02_1P80V_T (Dynamic_clamp), M3_PBIDIR_FS_DR_02_1P80V (I/O), M4_PBIDIR_FS_DR_02_1P80V (I/O), M4_PBIDIR_FS_DR_02_1P80V_T (Dynamic_clamp), M5_PBIDIR_FS_DR_02_1P80V (I/O), M5_PBIDIR_FS_DR_02_1P80V_T (Dynamic_clamp), M6_PBIDIR_FS_DR_04_1P80V (I/O), M7_PBIDIR_FS_DR_04_1P80V (I/O), M7_PBIDIR_FS_DR_04_1P80V_T (Dynamic_clamp), M8_PBIDIR_FS_DR_04_1P80V (I/O), M8_PBIDIR_FS_DR_04_1P80V_T (Dynamic_clamp), M9_PBIDIR_FS_DR_04_1P80V (I/O), M10_PBIDIR_FS_DR_0_1P80V (I/O), M10_PBIDIR_FS_DR_0_1P80V_T (Dynamic_clamp), M11_PBIDIR_FS_DR_0_1P80V (I/O), M11_PBIDIR_FS_DR_0_1P80V_T (Dynamic_clamp), M12_PBIDIR_FS_DR_0_1P80V (I/O)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
